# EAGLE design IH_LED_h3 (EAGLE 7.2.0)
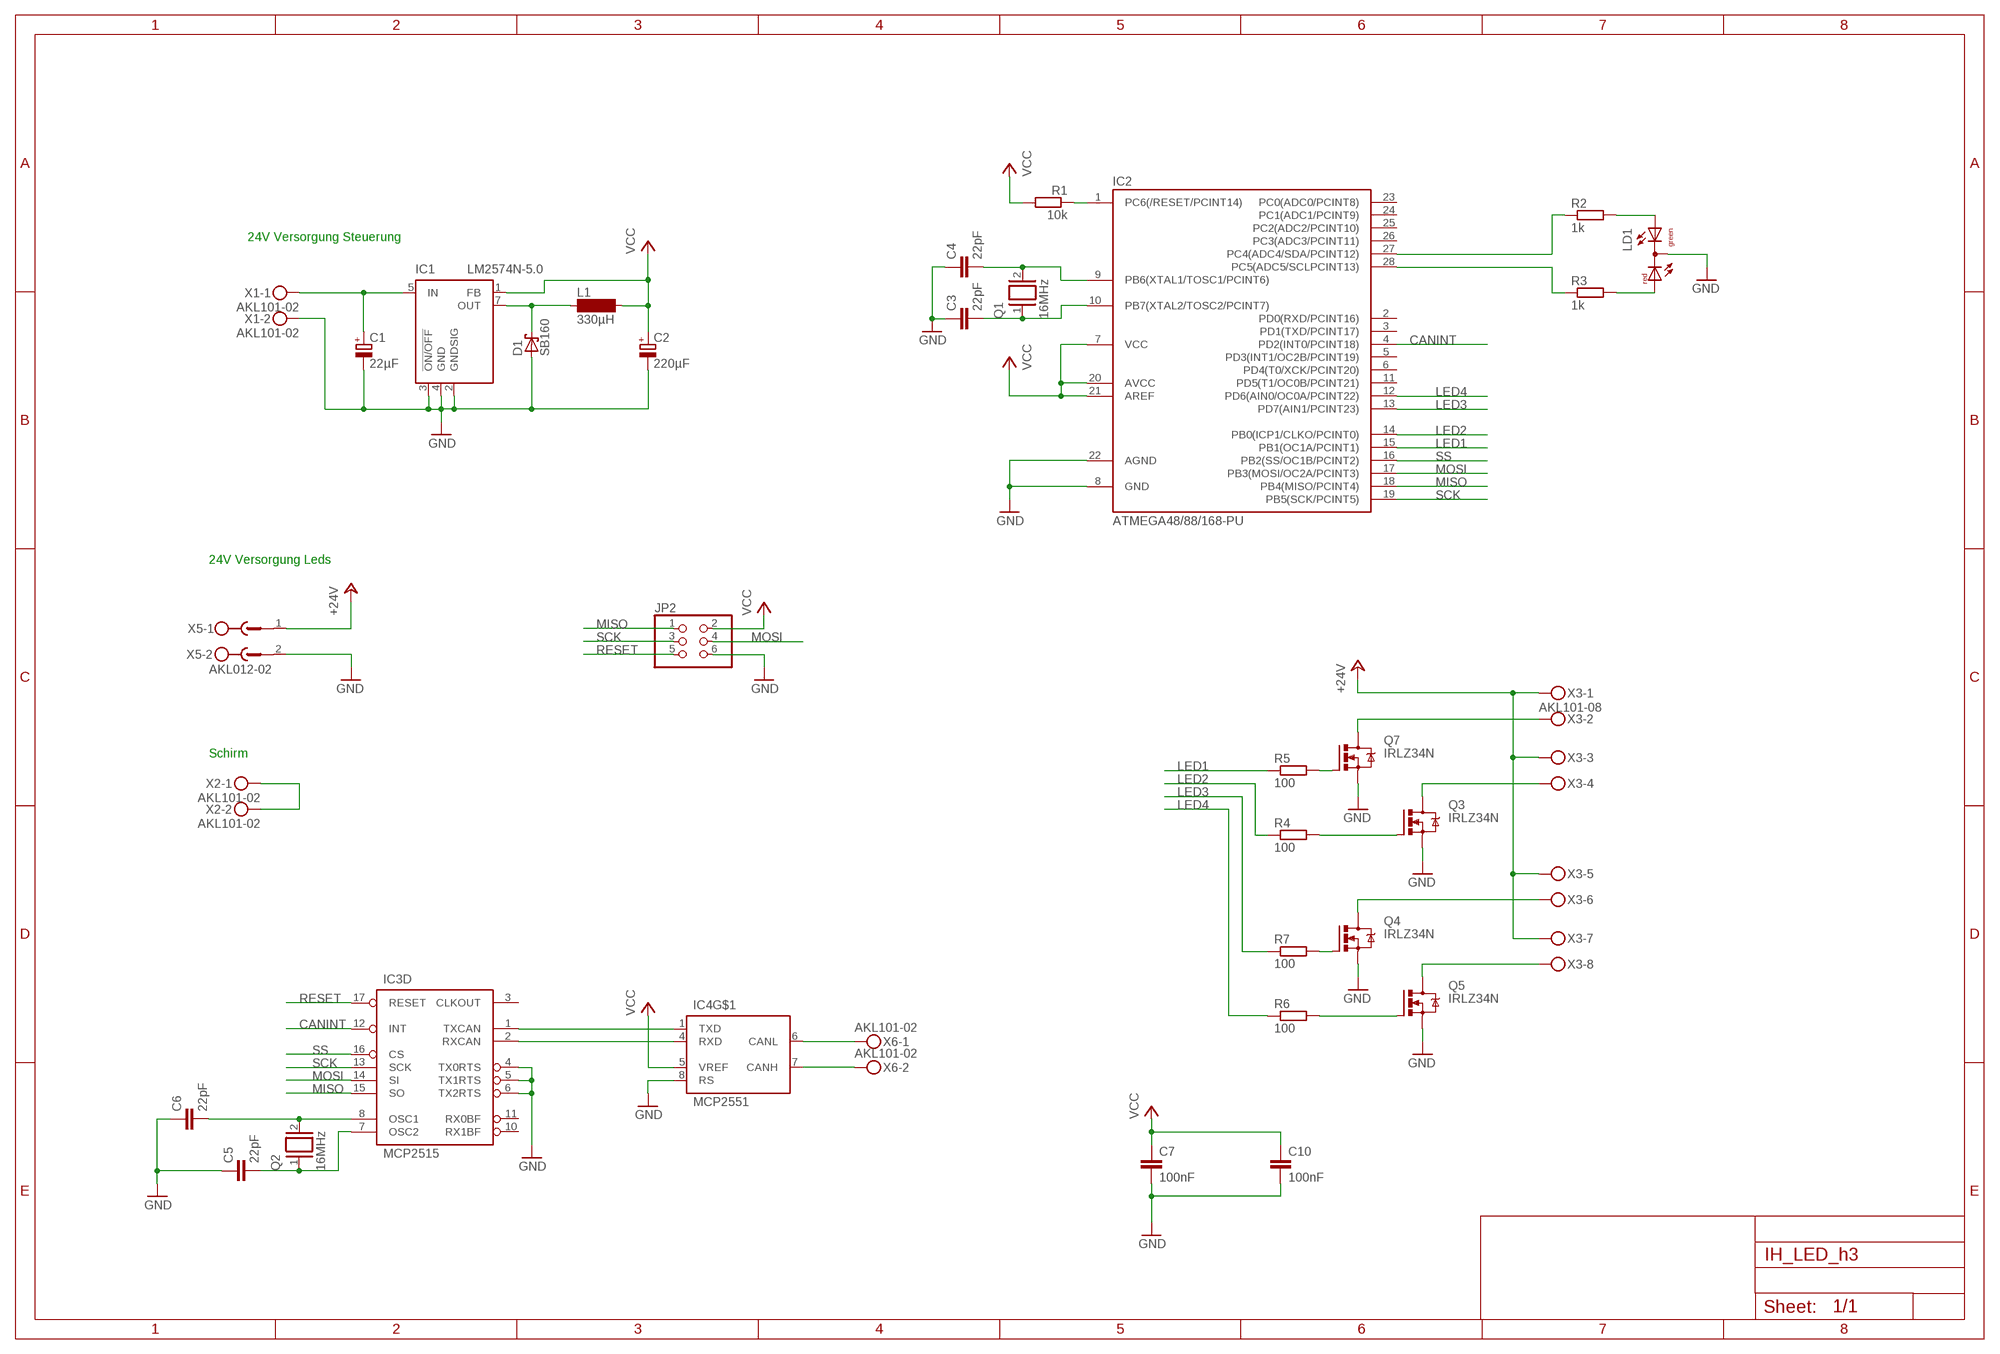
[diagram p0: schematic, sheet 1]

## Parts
C1  22µF  CPOL-EUE2-5  [E2-5]
C2  220µF  CPOL-EUE3.5-8  [E3,5-8]
C3  22pF  C-EUC0805  [C0805]
C4  22pF  C-EUC0805  [C0805]
C5  22pF  C-EUC0805  [C0805]
C6  22pF  C-EUC0805  [C0805]
C7  100nF  C-EUC0805  [C0805]
C10  100nF  C-EUC0805  [C0805]
D1  SB160  SCHOTTKY-DIODEDO35-7  [DO35-7]
IC1  LM2574N-5.0  [DIL08]
IC2  ATMEGA48/88/168-PU  [DIL28-3]
IC3  MCP2515  MCP2515P  [DIL18]
IC4  MCP2551  MCP2551DIL8  [DIL08]
JP2  PINHD-2X3  [2X03]
L1  330µH  SD12-1000  [SD12_1000]
LD1  DUOLED-RG-C  [DUOLED-C-5MM]
Q1  16MHz  XTAL/S  [QS]
Q2  16MHz  XTAL/S  [QS]
Q3  IRLZ34N  IRF530  [TO220BV]
Q4  IRLZ34N  IRF530  [TO220BV]
Q5  IRLZ34N  IRF530  [TO220BV]
Q7  IRLZ34N  IRF530  [TO220BV]
R1  10k  R-EU_M0805  [M0805]
R2  1k  R-EU_M0805  [M0805]
R3  1k  R-EU_M0805  [M0805]
R4  100  R-EU_0309/V  [0309V]
R5  100  R-EU_0309/V  [0309V]
R6  100  R-EU_0309/V  [0309V]
R7  100  R-EU_0309/V  [0309V]
X1  AKL101-02  MKDSN1,5/2-5,08  [MKDSN1,5/2-5,08]
X2  AKL101-02  MKDSN1,5/2-5,08  [MKDSN1,5/2-5,08]
X3  AKL101-08  MKDSN1,5/8-5,08  [MKDSN1,5/8-5,08]
X5  AKL012-02  MSTBV2  [MSTBV2]
X6  AKL101-02  MKDSN1,5/2-5,08  [MKDSN1,5/2-5,08]

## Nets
+24V: X3.1 X3.3 X3.5 X3.7 X5.1
CANINT: IC2.4(PD2(INT0/PCINT18)) IC3.12(D:INT)
GND: C1.- C2.- C3.1 C4.1 C5.1 C6.1 C7.2 C10.2 D1.A IC1.2(GNDSIG) IC1.3(!ON/OFF) IC1.4(GND) IC2.8(GND) IC2.22(AGND) IC3.4(D:TX0RTS) IC3.5(D:TX1RTS) IC3.6(D:TX2RTS) IC4.8(RS) JP2.6 LD1.C Q3.S Q4.S Q5.S Q7.S X1.2 X5.2
LED1: IC2.15(PB1(OC1A/PCINT1)) R5.1
LED2: IC2.14(PB0(ICP1/CLKO/PCINT0)) R4.1
LED3: IC2.13(PD7(AIN1/PCINT23)) R7.1
LED4: IC2.12(PD6(AIN0/OC0A/PCINT22)) R6.1
MISO: IC2.18(PB4(MISO/PCINT4)) IC3.15(D:SO) JP2.1
MOSI: IC2.17(PB3(MOSI/OC2A/PCINT3)) IC3.14(D:SI) JP2.4
N$1: IC3.1(D:TXCAN) IC4.1(TXD)
N$2: IC3.2(D:RXCAN) IC4.4(RXD)
N$3: C6.2 IC3.8(D:OSC1) Q2.2
N$4: C5.2 IC3.7(D:OSC2) Q2.1
N$5: IC4.6(CANL) X6.1
N$6: LD1.AX(AG) R2.2
N$7: C4.2 IC2.9(PB6(XTAL1/TOSC1/PCINT6)) Q1.2
N$8: C3.2 IC2.10(PB7(XTAL2/TOSC2/PCINT7)) Q1.1
N$9: IC4.7(CANH) X6.2
N$10: X2.1 X2.2
N$14: Q4.G R7.2
N$16: Q7.G R5.2
N$23: Q5.G R6.2
N$25: Q3.G R4.2
N$30: Q4.D X3.6
N$31: Q5.D X3.8
N$32: Q3.D X3.4
N$33: Q7.D X3.2
N$34: LD1.AR R3.2
N$35: C1.+ IC1.5(IN) X1.1
N$36: IC2.27(PC4(ADC4/SDA/PCINT12)) R2.1
N$37: IC2.28(PC5(ADC5/SCLPCINT13)) R3.1
N$76: D1.C IC1.7(OUT) L1.1
RESET: IC2.1(PC6(/RESET/PCINT14)) IC3.17(D:RESET) JP2.5 R1.1
SCK: IC2.19(PB5(SCK/PCINT5)) IC3.13(D:SCK) JP2.3
SS: IC2.16(PB2(SS/OC1B/PCINT2)) IC3.16(D:CS)
VCC: C2.+ C7.1 C10.1 IC1.1(FB) IC2.7(VCC) IC2.20(AVCC) IC2.21(AREF) IC4.5(VREF) JP2.2 L1.2 R1.2
Unconnected: IC2.2(PD0(RXD/PCINT16)) IC2.3(PD1(TXD/PCINT17)) IC2.5(PD3(INT1/OC2B/PCINT19)) IC2.6(PD4(T0/XCK/PCINT20)) IC2.11(PD5(T1/OC0B/PCINT21)) IC2.23(PC0(ADC0/PCINT8)) IC2.24(PC1(ADC1/PCINT9)) IC2.25(PC2(ADC2/PCINT10)) IC2.26(PC3(ADC3/PCINT11)) IC3.3(D:CLKOUT) IC3.10(D:RX1BF) IC3.11(D:RX0BF)

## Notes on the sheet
- 24V Versorgung Steuerung
- 24V Versorgung Leds
- Schirm

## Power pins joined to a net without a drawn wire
GND: IC3.9(P:GND) IC4.2(GND)
VCC: IC3.18(P:VCC) IC4.3(VCC)

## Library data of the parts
C1 C2 = rcl:CPOL-EU: POLARIZED CAPACITOR, European symbol
C3-C7 C10 = rcl:C-EU: CAPACITOR, European symbol
D1 = diode:SCHOTTKY-DIODE: Schottky Diode
IC1 = linear:LM2574?-*: SIMPLE SWITCHER 0.5A Step-Down Voltage Regulator Source: http://cache.national.com/ds/LM/LM2574.pdf
IC2 = atmega8:ATMEGA48/88/168-PU
IC3 = can:MCP2515: MC2515 Stand-Alone CAN Controller With SPI Interface, Microchip
IC4 = can:MCP2551: CAN Tranceiver Microchip
JP2 = pinhead:PINHD-2X3: PIN HEADER
L1 = inductor-neosid:SD12: INDUCTOR; OC_FARNELL: unknown; OC_NEWARK: unknown
LD1 = led:DUOLED-RG-C: DUO LED 2 colors (red/green), 5 mm, round, common Cathode www.ligitek.com or other producers.
Q1 Q2 = special:XTAL/S: CRYSTAL
Q3-Q5 Q7 = transistor-power:IRF530: HEXFET Power MOSFET
R1 = rcl:R-EU_: RESISTOR, European symbol
R2-R7 = resistor:R-EU_: RESISTOR, European symbol
X1 X2 X6 = con-phoenix-508:MKDSN1,5/2-5,08: MKDSN 1,5/ 2-5,08 Printklemme
X3 = con-phoenix-508:MKDSN1,5/8-5,08: MKDSN 1,5/ 8-5,08 Printklemme Nennstrom: 13,5 A Nennspannung: 250 V Rastermaß: 5,08 mm Polzahl: 8 Anschlussart: Schraubanschluss Montage: Löten Anschlussrichtung Leiter/Platine: 0 ° Artikelnummer: 1729186 Source: http://eshop.phoenixcontact.com .. 1729186.pdf
X5 = con-phoenix-500:MSTBV2: PHOENIX; OC_FARNELL: unknown; OC_NEWARK: unknown

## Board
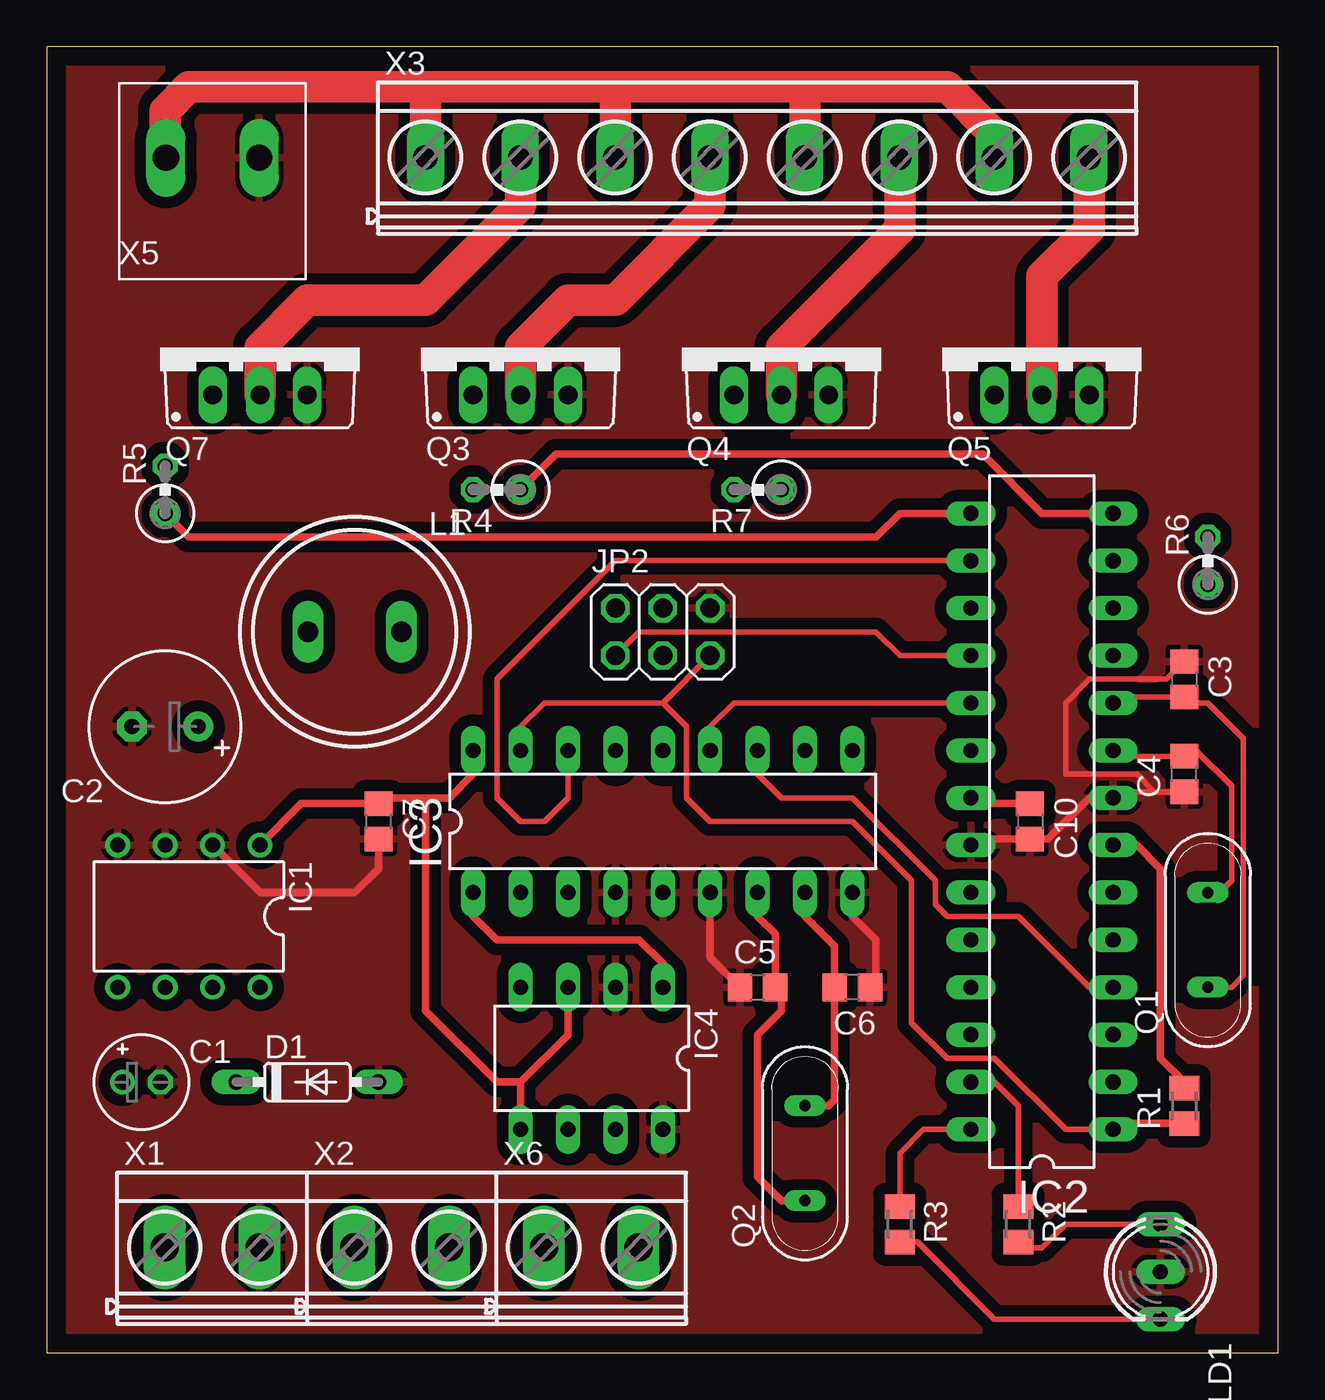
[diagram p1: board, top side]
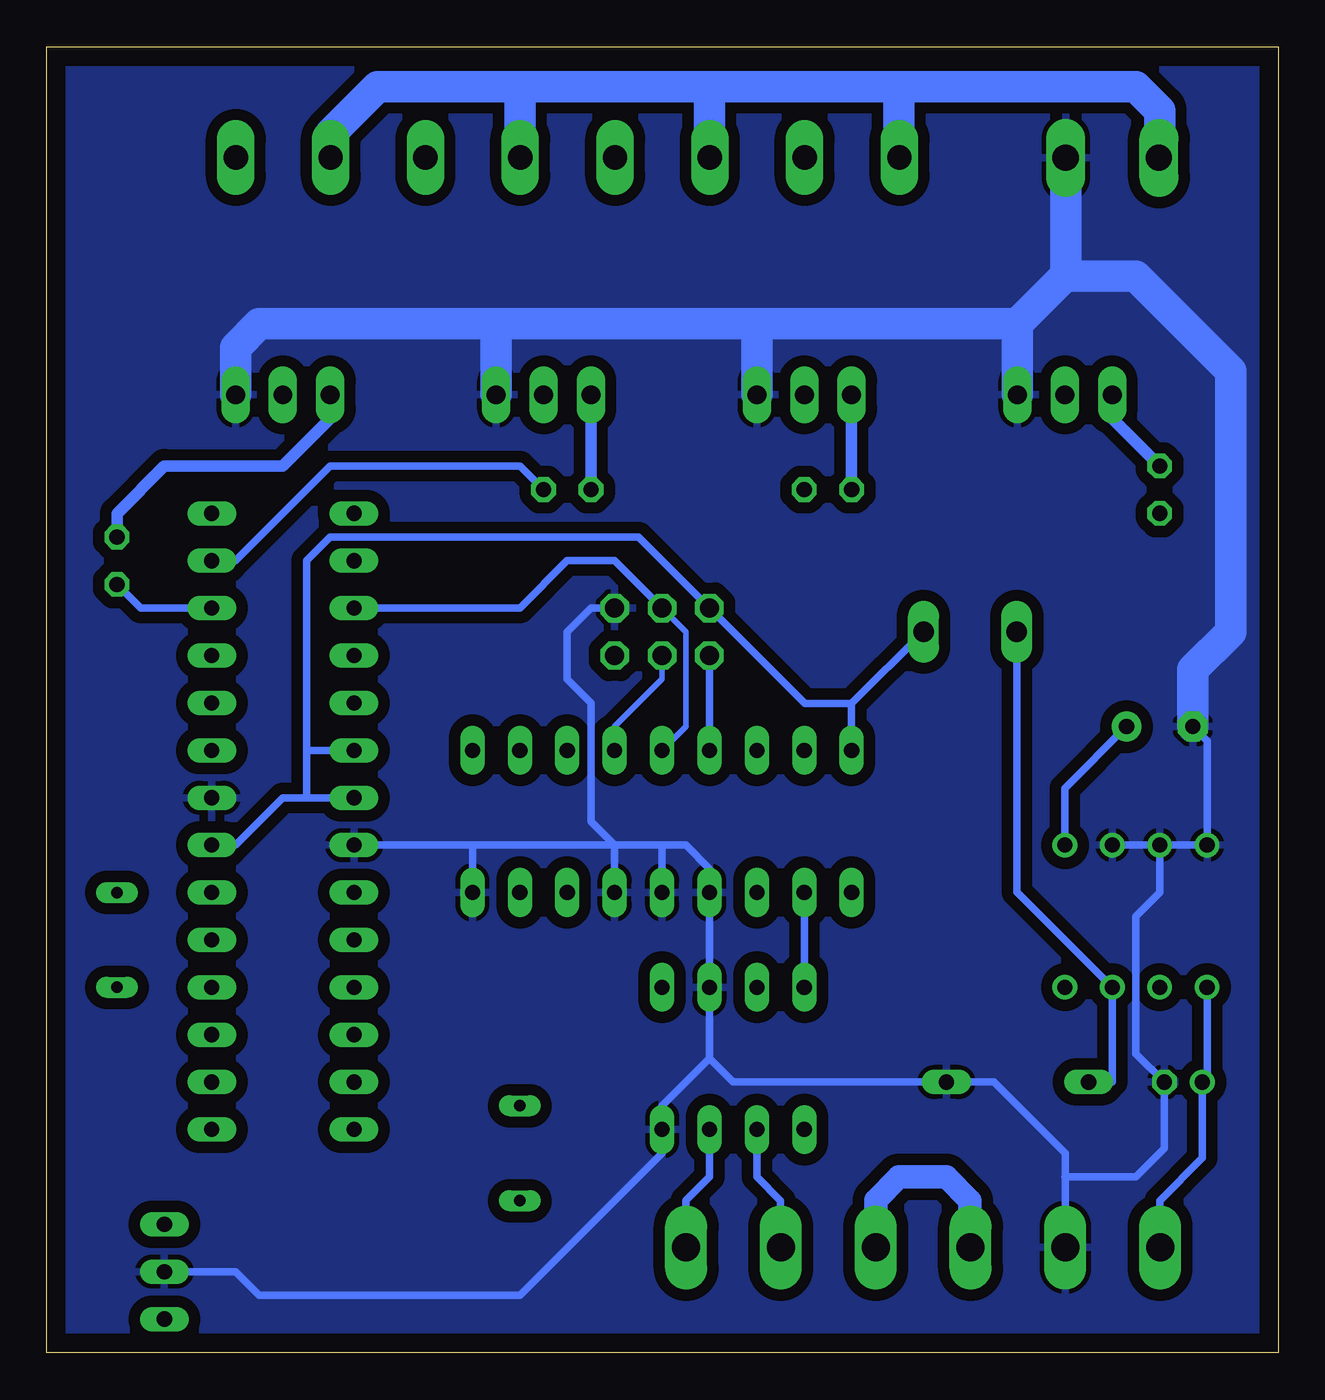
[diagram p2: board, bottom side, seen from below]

Size 66 x 70 mm. Coordinates in mm from the lower left corner, seen from the top.
Outline: 0,0 66,0 66,70 0,70 0,0
Copper layers (1*16): Top 0.035mm / dielectric 1.5mm / Bottom 0.035mm
Design rules "default": minimum track width 10mil, minimum drill 24mil, track to track 8mil, track to pad 8mil, pad to pad 8mil, via to via 8mil, smd to smd 8mil, copper to edge 40mil, drill to drill 8mil, minimum pad ring 10mil, minimum via ring 8mil, stop-mask expansion 4mil, vias tented up to drill 0mil, thermal gap 10mil

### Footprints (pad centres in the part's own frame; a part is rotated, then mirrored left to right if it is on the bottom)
E2-5 = drill 0.813 pad 1.27: + -1.016,0 | drill 0.813 pad 1.27 octagon: - 1.016,0
E3,5-8 = drill 0.813 pad 1.6: + -1.778,0 | drill 0.813 pad 1.6 octagon: - 1.778,0
C0805 = smd 1.3 x 1.5: 1 -0.95,0; 2 0.95,0
DO35-7 = drill 0.813 long: A 3.81,0; C -3.81,0
DIL08 = drill 0.813 pad 1.27: 1 -3.81,-3.81; 2 -1.27,-3.81; 3 1.27,-3.81; 4 3.81,-3.81; 5 3.81,3.81; 6 1.27,3.81; 7 -1.27,3.81; 8 -3.81,3.81
DIL28-3 = drill 0.813 long: 1 -16.51,-3.81; 2 -13.97,-3.81; 3 -11.43,-3.81; 4 -8.89,-3.81; 5 -6.35,-3.81; 6 -3.81,-3.81; 7 -1.27,-3.81; 8 1.27,-3.81; 9 3.81,-3.81; 10 6.35,-3.81; 11 8.89,-3.81; 12 11.43,-3.81; 13 13.97,-3.81; 14 16.51,-3.81; 15 16.51,3.81; 16 13.97,3.81; 17 11.43,3.81; 18 8.89,3.81; 19 6.35,3.81; 20 3.81,3.81; 21 1.27,3.81; 22 -1.27,3.81; 23 -3.81,3.81; 24 -6.35,3.81; 25 -8.89,3.81; 26 -11.43,3.81; 27 -13.97,3.81; 28 -16.51,3.81
DIL18 = drill 0.813 long: 1 -10.16,-3.81; 2 -7.62,-3.81; 3 -5.08,-3.81; 4 -2.54,-3.81; 5 0,-3.81; 6 2.54,-3.81; 7 5.08,-3.81; 8 7.62,-3.81; 9 10.16,-3.81; 10 10.16,3.81; 11 7.62,3.81; 12 5.08,3.81; 13 2.54,3.81; 14 0,3.81; 15 -2.54,3.81; 16 -5.08,3.81; 17 -7.62,3.81; 18 -10.16,3.81
DIL08' = drill 0.813 long: 1 -3.81,-3.81; 2 -1.27,-3.81; 3 1.27,-3.81; 4 3.81,-3.81; 5 3.81,3.81; 6 1.27,3.81; 7 -1.27,3.81; 8 -3.81,3.81
2X03 = drill 1.016 octagon: 1 -2.54,-1.27; 2 -2.54,1.27; 3 0,-1.27; 4 0,1.27; 5 2.54,-1.27; 6 2.54,1.27
SD12_1000 = drill 1.1 long: 1 -2.5,0; 2 2.5,0
DUOLED-C-5MM = drill 0.813 long: AR 2.54,0; AX -2.54,0; C 0,0
QS = drill 0.61 long: 1 -2.54,0; 2 2.54,0
TO220BV = drill 1.016 long: D 0,-2.54; G -2.54,-2.54; S 2.54,-2.54
M0805 = smd 1.3 x 1.6: 1 -0.95,0; 2 0.95,0
0309V = drill 0.813 octagon: 1 -1.27,0; 2 1.27,0
MKDSN1,5/2-5,08 = drill 1.5 long: 1 -2.561,0.025; 2 2.519,0.025
MKDSN1,5/8-5,08 = drill 1.3 pad 2 long: 1 -17.801,0.025; 2 -12.721,0.025; 3 -7.641,0.025; 4 -2.561,0.025; 5 2.519,0.025; 6 7.599,0.025; 7 12.679,0.025; 8 17.759,0.025
MSTBV2 = drill 1.4 long: 1 -2.5,0; 2 2.5,0

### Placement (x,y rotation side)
C1  5.08,14.51 0 top
C2  6.35,33.56 180 top
C3  60.96,36.1 270 top
C4  60.96,31.02 90 top
C5  38.1,19.59 0 top
C6  43.18,19.59 180 top
C7  17.78,28.48 270 top
C10  52.7,28.48 270 top
D1  13.97,14.51 0 top
IC1  7.62,23.4 180 top
IC2  53.34,28.48 90 top
IC3  33.02,28.48 0 top
IC4  MCP2551  [DIL08']  29.21,15.78 180 top
JP2  33.02,38.64 0 top
L1  16.51,38.64 0 top
LD1  59.69,4.35 270 top
Q1  62.23,22.13 90 top
Q2  40.64,10.7 90 top
Q3  25.4,53.88 0 top
Q4  39.37,53.88 0 top
Q5  53.34,53.88 0 top
Q7  11.43,53.88 0 top
R1  60.96,13.24 90 top
R2  52.07,6.89 270 top
R3  45.72,6.89 270 top
R4  24.13,46.26 180 top
R5  6.35,46.26 90 top
R6  62.23,42.45 90 top
R7  38.1,46.26 180 top
X1  8.89,5.62 0 top
X2  19.05,5.62 0 top
X3  38.1,64.04 0 top
X5  8.89,64.04 0 top
X6  29.21,5.62 0 top

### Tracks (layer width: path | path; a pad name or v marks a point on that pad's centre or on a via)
+24V
  Bottom 1.676: X5.1 6.35,64.08 6.35,66.58 7.62,67.85 20.32,67.85 | 20.32,67.85 30.48,67.85 | 30.48,67.85 40.64,67.85 | 40.64,67.85 48.26,67.85 50.78,65.33 X3.7 | X3.5 40.64,64.09 40.64,67.85 | X3.3 30.48,64.09 30.48,67.85 | X3.1 20.32,64.09 20.32,67.85
CANINT
  Top 0.305: IC3.12 38.1,31.02 39.37,29.75 43.18,29.75 47.62,25.3 47.62,24.04 48.26,23.4 52.07,23.4 55.88,19.59 IC2.4
GND
  Top 0.305: C3.1 60.01,36.1 55.88,36.1 54.61,34.83 54.61,31.02 58.42,31.02 59.37,30.07 C4.1 57.47,30.07 IC2.8
  Top 0.406: IC1.2 11.43,24.67 16.51,24.67 17.78,25.94 C7.2 | C5.1 35.56,21.18 IC3.6 | C6.1 44.45,19.91 44.45,22.13 43.18,23.4 IC3.9 | IC2.22 49.85,27.53 C10.2 53.66,27.53 55.88,29.75 IC2.8
  Bottom 0.406: IC1.3 6.35,24.67 7.62,23.4 7.62,16.03 C1.- 6.1,10.96 7.62,9.43 11.43,9.43 | IC1.3 IC1.4 3.81,32.8 C2.- | IC1.3 IC1.2 | 30.48,15.78 IC4.2 IC3.4 30.48,25.94 31.75,27.21 33.02,27.21 | 30.48,15.78 33.02,13.24 IC4.8 33.02,10.7 40.64,3.08 54.61,3.08 55.88,4.35 LD1.C | 30.48,15.78 29.21,14.51 D1.A 15.24,14.51 11.41,10.68 11.41,9.45 11.43,9.43 | 33.02,27.21 IC3.5 | IC3.6 35.56,27.21 | 35.56,27.21 33.02,27.21 | 35.56,27.21 36.83,28.48 36.83,34.83 38.1,36.1 38.1,38.64 36.83,39.91 JP2.6 | IC3.9 43.18,27.21 IC2.22 35.56,27.21 | 11.43,9.43 11.41,9.41 X1.2
  Bottom 1.676: Q7.S 13.97,55.15 | 13.97,55.15 27.94,55.15 | Q3.S 27.94,55.15 | 41.91,55.15 54.61,55.15 55.88,53.88 Q5.S | X5.2 11.39,57.73 11.43,57.69 | Q4.S 41.91,55.15 | 41.91,55.15 27.94,55.15 | 13.97,55.15 11.43,57.69 | 11.43,57.69 7.62,57.69 2.54,52.61 2.54,38.64 4.57,36.61 C2.-
  pour Bottom (isolate 0.61): -7.62,76.74 -7.62,-5.81 77.47,-5.81 77.47,76.74
  pour Top (isolate 0.61): -10.16,78.01 -10.16,-9.62 73.66,-9.62 73.66,78.01
LED1
  Top 0.406: IC2.15 45.72,44.99 44.45,43.72 7.62,43.72 R5.1
LED2
  Top 0.406: IC2.14 53.34,44.99 50.16,48.16 27.3,48.16 R4.1
LED3
  Bottom 0.406: IC2.13 55.88,42.45 50.8,47.53 40.64,47.53 R7.1
LED4
  Bottom 0.406: IC2.12 60.96,39.91 R6.1
MISO
  Top 0.305: JP2.1 31.75,38.64 44.45,38.64 45.72,37.37 IC2.18
  Bottom 0.406: IC3.15 JP2.1
MOSI
  Bottom 0.305: IC3.14 31.75,33.56 31.75,38.64 JP2.4
  Bottom 0.406: JP2.4 35.56,42.45 38.1,42.45 40.64,39.91 IC2.17
N$1
  Top 0.406: IC4.1 33.02,20.86 31.75,22.13 24.13,22.13 22.86,23.4 IC3.1
N$2
  Bottom 0.406: IC4.4 IC3.2
N$3
  Top 0.406: IC3.8 40.64,23.4 42.23,21.81 C6.2 42.23,13.56 41.91,13.24 Q2.2
N$4
  Top 0.406: IC3.7 38.1,23.4 39.05,22.45 C5.2 39.37,19.27 39.37,18.32 38.1,17.05 38.1,9.43 39.37,8.16 Q2.1
N$5
  Bottom 0.406: X6.1 26.67,5.67 26.67,8.16 27.94,9.43 IC4.6
N$6
  Top 0.305: R2.2 52.39,5.62 53.34,5.62 54.61,6.89 LD1.AX
N$7
  Top 0.305: IC2.9 57.47,31.97 C4.2 61.28,32.29 61.59,32.29 63.5,30.38 63.5,25.3 62.87,24.67 Q1.2
N$8
  Top 0.305: IC2.10 57.47,35.15 C3.2 61.28,34.83 62.23,34.83 64.14,32.92 64.14,20.23 63.5,19.59 Q1.1
N$9
  Bottom 0.406: IC4.7 30.48,9.43 31.73,8.18 X6.2
N$10
  Bottom 1.27: X2.1 16.51,5.67 16.51,8.16 17.78,9.43 20.32,9.43 21.57,8.18 X2.2
N$13
  Top 1.676: 6.35,64.04 6.35,66.58 7.62,67.85 20.32,67.85 | 20.32,67.85 30.48,67.85 | 30.48,67.85 40.64,67.85 | 40.64,67.85 48.26,67.85 50.8,65.31 50.8,64.04 | 20.32,64.04 20.32,67.85 | 30.48,64.04 30.48,67.85 | 40.64,64.04 40.64,67.85
N$14
  Bottom 0.61: R7.2 Q4.G
N$16
  Bottom 0.61: R5.2 8.89,50.07 Q7.G
N$23
  Bottom 0.61: R6.2 62.23,44.99 59.69,47.53 53.34,47.53 50.8,50.07 Q5.G
N$25
  Bottom 0.61: R4.2 Q3.G
N$30
  Top 1.676: Q4.D 39.37,53.88 45.72,60.23 45.72,64.04 X3.6
N$31
  Top 1.676: Q5.D 53.34,57.69 55.88,60.23 55.88,64.04 X3.8
N$32
  Top 1.676: Q3.D 25.4,53.88 27.94,56.42 30.48,56.42 35.56,61.5 35.56,64.04 X3.4
N$33
  Top 1.676: Q7.D 11.43,53.88 13.97,56.42 20.32,56.42 25.4,61.5 25.4,64.04 X3.2
N$34
  Top 0.305: LD1.AR 50.8,1.81 46.67,5.94 R3.2
N$35
  Bottom 0.406: IC1.5 3.81,14.76 C1.+ 4.06,10.45 6.35,8.16 6.35,5.67 X1.1
N$36
  Top 0.305: IC2.27 50.8,14.51 52.07,13.24 R2.1
N$37
  Top 0.305: IC2.28 46.99,11.97 45.72,10.7 R3.1
N$76
  Bottom 0.406: D1.C 8.89,14.51 IC1.7 14.01,24.71 L1.1
RESET
  Top 0.305: JP2.5 33.02,34.83 | 33.02,34.83 26.67,34.83 25.4,33.56 IC3.17 | 33.02,34.83 34.29,33.56 34.29,29.75 35.56,28.48 43.18,28.48 46.35,25.3 46.35,17.68 48.26,15.78 50.8,15.78 54.61,11.97 IC2.1
  Top 0.406: IC2.1 57.47,12.29 R1.1
SCK
  Top 0.305: IC2.19 36.83,34.83 35.56,33.56 IC3.13
  Bottom 0.305: IC3.13 35.56,33.56 33.02,36.1 JP2.3
SS
  Top 0.305: IC2.16 30.48,42.45 24.13,36.1 24.13,29.75 25.4,28.48 26.67,28.48 27.94,29.75 IC3.16
VCC
  Top 0.406: IC1.1 13.65,29.43 C7.1 18.1,29.75 20.32,29.75 | IC3.18 22.86,31.02 21.59,29.75 20.32,29.75 | IC4.5 25.4,14.51 | 25.4,14.51 27.94,17.05 IC4.3 | 25.4,14.51 24.13,14.51 20.32,18.32 20.32,29.75 | IC2.21 49.85,29.43 C10.1 | IC2.7 58.42,27.21 59.69,25.94 59.69,15.78 60.96,14.51 R1.2
  Bottom 0.406: C2.+ 11.43,30.26 IC1.1 | L1.2 22.86,34.79 | 22.86,34.79 IC3.18 | 22.86,34.79 25.36,34.79 JP2.2 34.29,43.72 50.8,43.72 52.07,42.45 52.07,32.29 | IC2.7 55.88,27.21 53.34,29.75 52.07,29.75 | 52.07,29.75 IC2.21 | IC2.20 52.07,32.29 | 52.07,32.29 52.07,29.75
